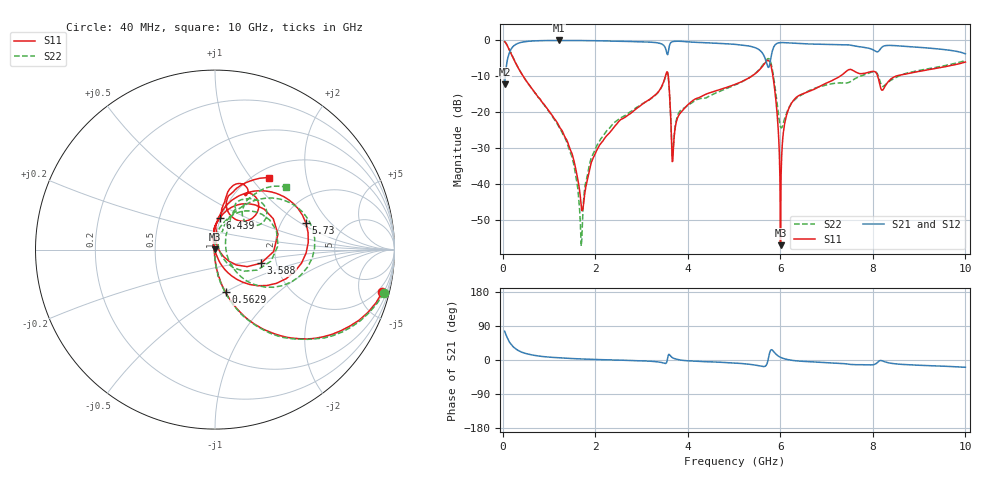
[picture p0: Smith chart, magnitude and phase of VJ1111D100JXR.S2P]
! VJ1111D100JXR
! DATE 03/04/2022  14:25
! CAPACITORS MOUNTED IN SERIES ON 25 MIL THICK MICROSTRIP SUBSTRATE
# GHz  S  MA  R  50.00
!  FREQ  S11M  S11A  S21M  S21A  S12M  S12A  S22M  S22A
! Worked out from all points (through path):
!   801 points, 40 MHz to 10 GHz, reference 50 ohm
!   highest |S21| = -0.01 dB at 1.21 GHz (marker M1); lowest = -12.2 dB at 40 MHz (marker M2)
!   group delay of S21, straight-line fit = 8.58 ps
!   lowest |S11| = -56.9 dB at 6.004 GHz (marker M3), VSWR 1.00, Z = 49.9 + j0.0641 ohm
!   |S11| at or under -10 dB: 443.2 MHz to 3.515 GHz (3.072 GHz wide, 155 % of centre); 3.578 GHz to 5.375 GHz (1.797 GHz wide, 40.1 % of centre); 5.841 GHz to 7.284 GHz (1.443 GHz wide, 22 % of centre)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
!   |S22| runs from -57.2 to -0.2 dB; largest |S21 - S12| = 0.013
!   S11 on the Smith chart (normalised r, x): 40 MHz: 1.23, -7.84; 562.9 MHz: 1.00, -0.50; 3.588 GHz: 1.66, -0.27; 5.73 GHz: 2.72, +1.11; 6.439 GHz: 0.99, +0.36; 10 GHz: 1.16, +1.23
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0.04  0.9623 -14.2  0.2448 75.8  0.2455 75.8  0.9724 -14.5
0.2641  0.5048 -59.7  0.8668 31.2  0.867 30.6  0.5079 -59.9
0.5629  0.2445 -76.1  0.9739 15.2  0.9773 15.2  0.2444 -76.7
1.2103  0.06565 -88.6  0.999 5.7  1.003 5.6  0.06347 -88.8
1.5091  0.02509 -95.8  0.9974 3.8  1.002 3.7  0.02252 -95.0
1.7083  0.004306 -159.9  0.9952 2.7  1 2.6  0.001712 140.5
1.84525  0.01268 109.6  0.9931 2.1  0.9974 2.0  0.01507 93.5
2.0818  0.03427 99.2  0.9881 1.1  0.9925 1.0  0.03934 87.9
3.36415  0.1934 78.9  0.9203 -5.2  0.9247 -5.3  0.1918 67.0
3.58825  0.2677 -16.4  0.7597 14.9  0.7629 14.8  0.2618 -25.8
3.68785  0.03116 71.7  0.9676 4.9  0.9711 4.7  0.03342 57.6
4.01155  0.1297 88.4  0.9536 -2.3  0.9568 -2.3  0.1257 69.3
5.02  0.2446 76.5  0.8818 -8.0  0.8853 -8.1  0.2404 61.8
5.72965  0.5275 16.2  0.4311 -2.5  0.4323 -2.8  0.5572 11.2
5.8666  0.2391 -49.5  0.8312 20.7  0.8345 20.5  0.2752 -43.1
6.00355  0.001431 153.3  0.9319 7.1  0.9354 7.0  0.06291 -7.7
6.15295  0.1001 93.4  0.9274 1.3  0.9309 1.2  0.1052 53.3
6.4393  0.1763 81.0  0.9011 -3.2  0.9043 -3.3  0.1719 61.6
6.6883  0.2033 80.1  0.8911 -4.9  0.8939 -5.0  0.2089 63.9
7.49755  0.395 68.0  0.8628 -11.4  0.8659 -11.5  0.2635 65.0
8.34415  0.2727 76.6  0.853 -7.5  0.8573 -7.5  0.2667 55.1
10  0.5007 53.0  0.6506 -19.2  0.6536 -19.4  0.5245 41.5
